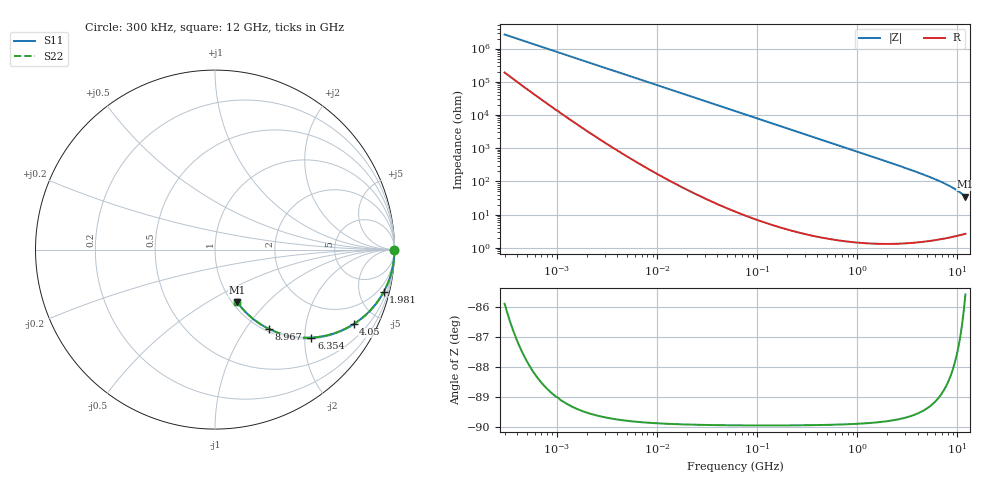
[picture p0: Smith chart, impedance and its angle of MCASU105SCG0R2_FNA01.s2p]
! MCASU105SCG0R2_FNA01  S-PARAMETER MODEL  ( Standard Model )
! Model Generated by TAIYO YUDEN Corporation (http://www.ty-top.com)
! Version 1.0
! TAIYO YUDEN Control No. 230609
! Copyright(c) 2023 TAIYO YUDEN CO.,LTD. All Rights Reserved.
! Product Description (link to TY-COMPAS)
! https://ds.yuden.co.jp/TYCOMPAS/or/detail?pn=MCASU105SCG0R2CFNA01&u=M
! Products Name : Multilayer Ceramic Capacitors
! Characteristics :
!  Capacitance : 0.2 [pF] , Rated Voltage : 50 [V] , TCC : CG / C0G
!  Case Size : 1.0 x 0.5 / 0.039 x 0.02 [mm/inch] , Thickness : 0.5 / 0.02 [mm/inch]
!  (Conditions: Temperature = 25 [degC] , DC Bias Voltage = 0 [V])
! External Node Assignments :
!  1  o---| |---o  2
! GND o---------o GND
! Frequency Range : 0.3MHz  -  12000MHz  [ 401 STEP ]
# MHZ S RI R 50
! Freq[MHz].  S11 Real  S11 Imag  S21 Real  S21 Imag  S12 Real  S12 Imag  S22 Real  S22 Imag
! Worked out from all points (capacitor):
!   401 points, 300 kHz to 12 GHz, reference 50 ohm
!   read as one part in series: C = 201 fF near 316.3 kHz
!   lowest |Z| = 34.6 ohm at 12 GHz (marker M1)
!   S11 on the Smith chart (normalised r, x): 300 kHz: open; 1.981 GHz: 1.03, -7.89; 4.05 GHz: 1.03, -3.70; 6.354 GHz: 1.04, -2.16; 8.967 GHz: 1.04, -1.30; 12 GHz: 1.05, -0.69
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0.3  1 -3.77e-05  2.7e-06 3.77e-05  2.7e-06 3.77e-05  1 -3.77e-05
0.778586  1 -9.83e-05  2.24e-06 9.83e-05  2.24e-06 9.83e-05  1 -9.83e-05
0.842989  1 -0.000106  2.22e-06 0.000106  2.22e-06 0.000106  1 -0.000106
1.769972  1 -0.000224  2.14e-06 0.000224  2.14e-06 0.000224  1 -0.000224
10.44266  1 -0.00132  4.46e-06 0.00132  4.46e-06 0.00132  1 -0.00132
60  0.9999 -0.00758  6.45e-05 0.00758  6.45e-05 0.00758  0.9999 -0.00758
164.1901  0.9996 -0.0207  0.000448 0.0207  0.000448 0.0207  0.9996 -0.0207
353.9943  0.998 -0.0446  0.00204 0.0446  0.00204 0.0446  0.998 -0.0446
585.5907  0.9945 -0.0736  0.00555 0.0736  0.00555 0.0736  0.9945 -0.0736
918.7169  0.9864 -0.1148  0.0136 0.1148  0.0136 0.1148  0.9864 -0.1148
1366.97  0.9703 -0.1685  0.0297 0.1685  0.0297 0.1685  0.9703 -0.1685
1980.756  0.9389 -0.2378  0.0611 0.2378  0.0611 0.2378  0.9389 -0.2378
2088.533  0.9324 -0.2493  0.0676 0.2493  0.0676 0.2493  0.9324 -0.2493
2947.191  0.8706 -0.333  0.1294 0.333  0.1294 0.333  0.8706 -0.333
4050.141  0.7719 -0.4157  0.2281 0.4157  0.2281 0.4157  0.7719 -0.4157
5006.236  0.676 -0.4626  0.324 0.4626  0.324 0.4626  0.676 -0.4626
6354.153  0.5376 -0.4905  0.4624 0.4905  0.4624 0.4905  0.5376 -0.4905
7648.807  0.4127 -0.4808  0.5873 0.4808  0.5873 0.4808  0.4127 -0.4808
8966.534  0.3019 -0.4428  0.6981 0.4428  0.6981 0.4428  0.3019 -0.4428
9968.853  0.2312 -0.4005  0.7688 0.4005  0.7688 0.4005  0.2312 -0.4005
10793.46  0.1821 -0.3597  0.8179 0.3597  0.8179 0.3597  0.1821 -0.3597
12000  0.1249 -0.2943  0.8751 0.2943  0.8751 0.2943  0.1249 -0.2943
